FUNCTION_BLOCK "FB_Average"
TITLE =Funktionsbaustein zur laufenden Mittelwertberechnung
VERSION : 0.1


VAR_INPUT
  RESET : BOOL ;	//Rücksetzen/ Initalisieren des Mittelwerts
  VALUE : REAL ;	//Von diesem Wert soll der laufende Mitetlwert berechnet werden
  BY_VALUE_CHANGE : BOOL  := TRUE;	//TRUE: neuer MW nur bei Änderung von VALUE,FALSE: neuer MW bei jedem Zyklus
END_VAR
VAR_OUTPUT
  AVERAGE : REAL ;	//Rückgabeausgang für den laufenden Mittelwert
END_VAR
VAR
  Anzahl : REAL ;	//Anzahl bisher eingerechnete Werte
  Aktueller_Mittelwert : REAL ;	//Aktueller Mittelwert
  OldValue : REAL ;
END_VAR
VAR_TEMP
  Resultat : REAL ;
END_VAR
BEGIN
NETWORK
TITLE =Rücksetzanforderung bearbeiten

      U     #RESET;
      SPBNB _001;
      L     0;
      T     #Anzahl;
      L     0.000000e+000;
      T     #Aktueller_Mittelwert;
      T     #OldValue;
      T     #AVERAGE;
      BEB   ;
_001: NOP   0;
NETWORK
TITLE =Mittelwert berechnen

// Berechnungsmodus abfragen
// Wenn BY_VALUE_CHANGE = FALSE, den Mittelwert
// bei jedem Aufruf berechnen, ansonsten nur wenn
// der Eingangswert sich ändert
      UN    #BY_VALUE_CHANGE;
      SPB   nmw;

//
// Eingangswert abfragen
//
      L     #OldValue;
      L     #VALUE;
      ==R   ;
      BEB   ;

//
// Zwischenspeichern von Eingangswert, wenn er sich
// geändert hat
//
      L     #VALUE;
      T     #OldValue;

//
// Mittelwert berechnen
//
nmw:  L     #Anzahl;
      L     #Aktueller_Mittelwert;
      *R    ;
      L     #VALUE;
      +R    ;
      T     #Resultat;
// Anzahl um eins erhöhen
      L     #Anzahl;
      L     1.000000e+000;
      +R    ;
      T     #Anzahl;
// Neuen Mittelwert berechnen
      L     #Resultat;
      L     #Anzahl;
      /R    ;
      T     #Aktueller_Mittelwert;
      T     #AVERAGE;
      BE    ;
END_FUNCTION_BLOCK

